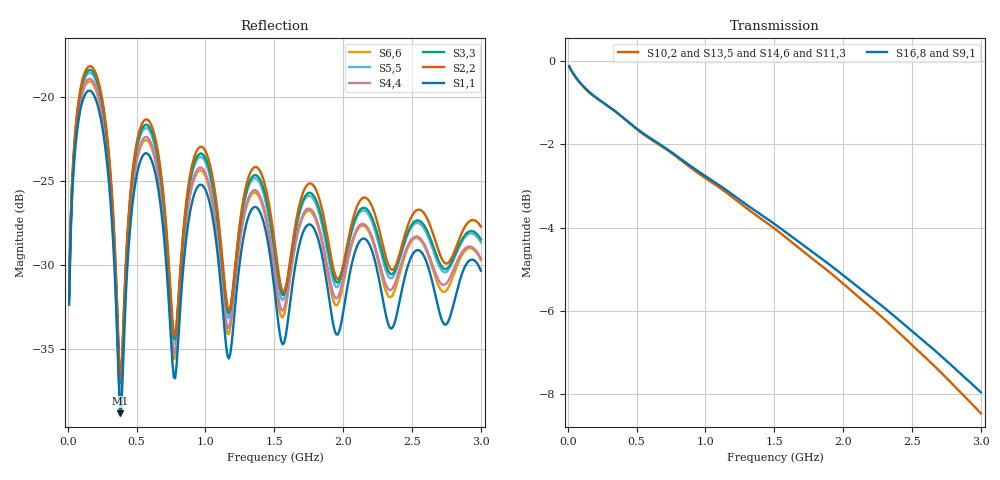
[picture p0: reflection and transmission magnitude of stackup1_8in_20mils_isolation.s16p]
! Touchstone file from project
# GHZ S RI R 50.000000
! Modal data exported
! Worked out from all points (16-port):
!   300 points, 10 MHz to 3 GHz, reference 50 ohm
!   strongest paths, dB at 10 MHz, 760 MHz, 1.51 GHz, 2.26 GHz, 3 GHz:
!     S16,8: -0.1, -2.2, -3.9, -5.8, -8.0
!     S9,1: -0.1, -2.2, -4.0, -5.9, -8.0
!     S10,2: -0.1, -2.2, -4.0, -6.1, -8.5
!     S13,5: -0.1, -2.2, -4.1, -6.1, -8.5
!     S14,6: -0.1, -2.2, -4.1, -6.1, -8.5
!     S11,3: -0.1, -2.2, -4.1, -6.1, -8.5
!   lowest |S11| = -38.8 dB at 380 MHz (marker M1), VSWR 1.02, Z = 51 - j0.591 ohm
!   |S11| at or under -10 dB: start of sweep to end of sweep
